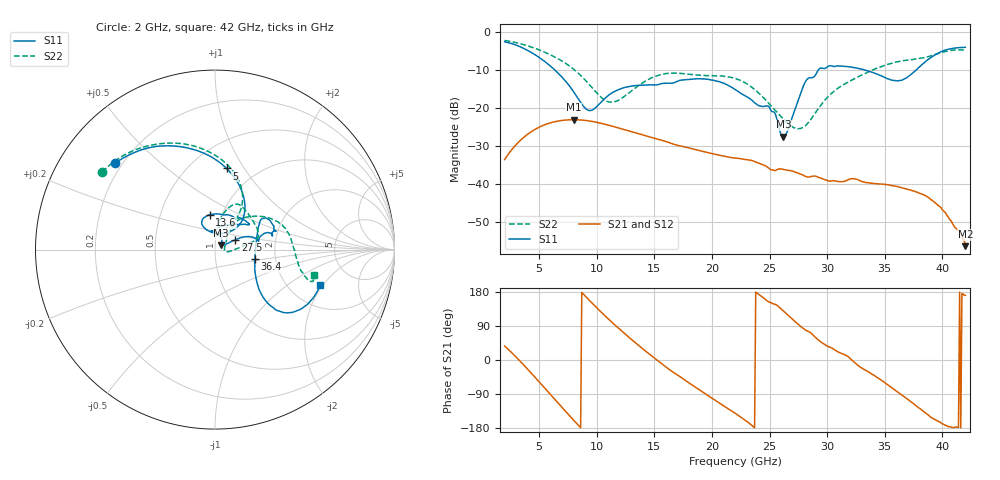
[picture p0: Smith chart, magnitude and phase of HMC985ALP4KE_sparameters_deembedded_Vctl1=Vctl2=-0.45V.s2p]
!s2p File: Measurements: S11, S21, S12, S22
# GHz S dB R 50.0
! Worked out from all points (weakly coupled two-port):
!   401 points, 2 GHz to 42 GHz, reference 50 ohm
!   highest |S21| = -23.18 dB at 8 GHz (marker M1); lowest = -56.4 dB at 42 GHz (marker M2)
!   lowest |S11| = -27.7 dB at 26.2 GHz (marker M3), VSWR 1.09, Z = 53.5 + j2.49 ohm
!   |S11| at or under -10 dB: 6.319 GHz to 29.27 GHz (22.95 GHz wide, 129 % of centre); 33.14 GHz to 37.77 GHz (4.624 GHz wide, 13 % of centre)
!   |S22| runs from -25.6 to -2.3 dB; largest |S21 - S12| = 0.00018
!   S11 on the Smith chart (normalised r, x): 2 GHz: 0.17, +0.36; 5 GHz: 0.73, +0.84; 13.6 GHz: 0.88, +0.35; 27.5 GHz: 1.25, +0.14; 36.4 GHz: 1.56, -0.17; 42 GHz: 2.94, -1.89
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2  -2.67 139.0  -33.68 37.0  -33.69 37.1  -2.35 145.5
3.4  -4.08 112.5  -28.54 -4.8  -28.54 -4.8  -3.23 123.1
5  -6.81 81.8  -25.15 -57.8  -25.16 -57.8  -4.83 98.6
8  -15.88 46.1  -23.18 -159.1  -23.19 -159.1  -9.93 61.1
8.7  -19.08 56.7  -23.28 178.3  -23.28 178.3  -11.84 56.8
9.6  -20.64 91.9  -23.64 150.0  -23.64 150.0  -14.78 55.9
11.1  -16.60 117.4  -24.70 105.5  -24.70 105.6  -18.55 71.1
13.6  -14.15 98.6  -26.84 39.3  -26.85 39.3  -14.27 78.2
15.4  -13.90 73.7  -28.40 -3.9  -28.40 -3.9  -11.46 68.3
19.4  -12.51 36.2  -31.67 -88.7  -31.68 -88.7  -11.57 34.8
22  -15.20 53.5  -33.27 -140.3  -33.28 -140.3  -12.34 14.7
24.9  -19.63 97.3  -35.85 153.8  -35.85 153.8  -18.78 1.2
26.2  -27.68 34.3  -36.26 128.9  -36.26 128.9  -23.02 -9.9
27.5  -18.01 25.8  -37.27 93.7  -37.28 93.8  -25.55 0.9
28.1  -13.26 18.9  -38.08 79.3  -38.02 79.4  -24.79 18.9
28.7  -12.12 11.4  -38.05 68.2  -38.04 68.3  -22.59 34.4
31  -9.05 22.0  -39.44 20.6  -39.48 20.5  -14.76 53.7
33.3  -10.14 33.3  -39.68 -26.3  -39.67 -26.3  -11.04 41.2
35.4  -12.56 11.7  -40.39 -68.5  -40.41 -68.7  -8.53 25.3
36.4  -12.86 -13.5  -41.00 -90.5  -41.05 -90.7  -7.76 16.9
39.5  -5.92 -43.2  -45.32 -159.9  -45.38 -159.3  -5.89 -14.9
42  -4.15 -18.6  -56.44 171.1  -56.31 167.7  -4.93 -14.4
